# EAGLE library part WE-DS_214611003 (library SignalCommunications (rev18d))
WE-DS D-SUB-Filter, Solder Pin Straight Characteristics Standard type filtered with 1000 pF High attenuation: max. ≥ 40 dB @ 180 MHz Choice of UNC 4/40 or through hole Rated voltage: 100 VDC Rated current @ 20 ºC: 5 A Withstand voltage: 250 VRMS Insulation resistance: min. 1000 MΩ Operating temperature: –55 ºC to +125 ºC Applications Filtering of interfaces External connection to -printer -sensor -display Details see: http://katalog.we-online.de/en/pbs/Filter_gerade Created on 2015-05-04 2015 (C) Wurth Elektronik
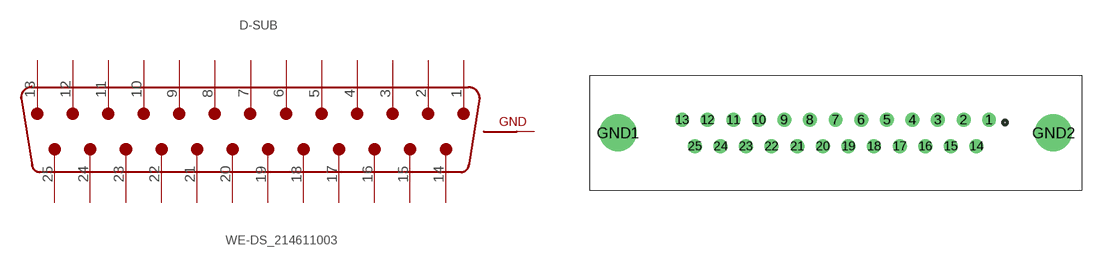
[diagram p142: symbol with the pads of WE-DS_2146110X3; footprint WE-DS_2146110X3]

Designator prefix D-SUB

## WE-DS_214611003 (WE-NUMBER: 214611003/25 pins_female)  [WE-DS_2146110X3]
1  13  pas
2  12  pas
3  11  pas
4  10  pas
5  9  pas
6  8  pas
7  7  pas
8  6  pas
9  5  pas
10  4  pas
11  3  pas
12  2  pas
13  1  pas
14  25  pas
15  24  pas
16  23  pas
17  22  pas
18  21  pas
19  20  pas
20  19  pas
21  18  pas
22  17  pas
23  16  pas
24  15  pas
25  14  pas
GND1  GND  pwr
GND2  GND  pwr

## Footprint WE-DS_2146110X3 (pad centres in mm)
drill 1: 1 16.56,1.42; 2 13.82,1.42; 3 11.05,1.42; 4 8.28,1.42; 5 5.54,1.42; 6 2.77,1.42; 7 0,1.42; 8 -2.77,1.42; 9 -5.54,1.42; 10 -8.28,1.42; 11 -11.05,1.42; 12 -13.82,1.42; 13 -16.56,1.42; 14 15.19,-1.42; 15 12.42,-1.42; 16 9.68,-1.42; 17 6.91,-1.42; 18 4.14,-1.42; 19 1.38,-1.42; 20 -1.38,-1.42; 21 -4.14,-1.42; 22 -6.91,-1.42; 23 -9.68,-1.42; 24 -12.42,-1.42; 25 -15.19,-1.42
drill 3: GND1 -23.5,0; GND2 23.5,0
